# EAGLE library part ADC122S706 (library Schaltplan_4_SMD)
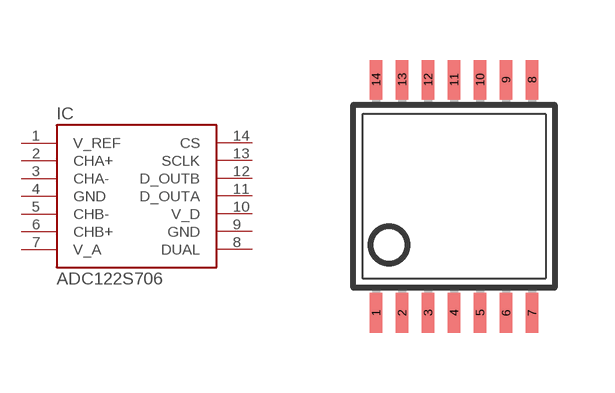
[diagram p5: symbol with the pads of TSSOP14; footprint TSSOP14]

Designator prefix IC

## ADC122S706  [TSSOP14]
1  V_REF
2  CHA+
3  CHA-
4  GND
5  CHB-
6  CHB+
7  V_A
8  DUAL
9  GND
10  V_D
11  D_OUTA
12  D_OUTB
13  SCLK
14  CS

## Footprint TSSOP14 (pad centres in mm)
Thin Shrink Small Outline Plastic 14 MAX3223-MAX3243.pdf
smd 0.305 x 0.991: 1 -1.95,-2.918; 2 -1.3,-2.918; 3 -0.65,-2.918; 4 0,-2.918; 5 0.65,-2.918; 6 1.3,-2.918; 7 1.95,-2.918; 8 1.95,2.918; 9 1.3,2.918; 10 0.65,2.918; 11 0,2.918; 12 -0.65,2.918; 13 -1.3,2.918; 14 -1.95,2.918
